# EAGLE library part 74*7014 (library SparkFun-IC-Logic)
Schmitt-trigger Hex Buffer The 74HC7014 is a hex buffer with precision Schmitt-trigger inputs. The precisely defined trigger levels are lying in a window between (0.55 x VCC) and (0.65 x VCC). It makes the circuit suitable to operate in a highly noisy environment. Input shorts are allowed to -1.5 V and +16 V without disturbing other channels. Inputs include clamp diodes that enable the use of current limiting resistors to interface inputs to voltages in excess of VCC. Schmitt trigger inputs transform slowly changing input signals into sharply defined jitter-free output signals. SparkFun Products SparkFun Stepoko (ROB-13899)
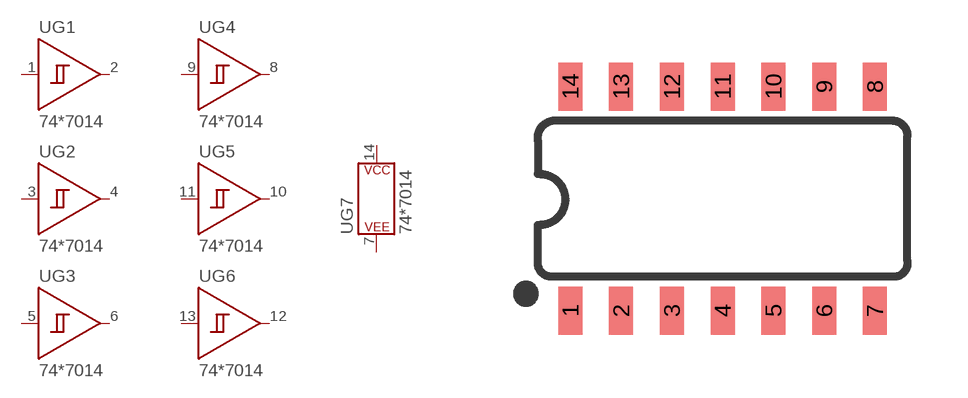
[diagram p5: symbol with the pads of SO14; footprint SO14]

Designator prefix U; gates G1=GATE_INVERTER_SCHMITT_TRIGGER G2=GATE_INVERTER_SCHMITT_TRIGGER G3=GATE_INVERTER_SCHMITT_TRIGGER G4=GATE_INVERTER_SCHMITT_TRIGGER G5=GATE_INVERTER_SCHMITT_TRIGGER G6=GATE_INVERTER_SCHMITT_TRIGGER G7=POWER_CONSORT

## 74HC7014D (PROD_ID: IC-12527; VALUE: 74HC7014D)  [SO14]
1  G1:A
2  G1:Y
3  G2:A
4  G2:Y
5  G3:A
6  G3:Y
7  G7:P$V-
8  G4:Y
9  G4:A
10  G5:Y
11  G5:A
12  G6:Y
13  G6:A
14  G7:P$V+

## Footprint SO14 (pad centres in mm)
SOIC, 0.15 inch width
smd 0.6 x 1.2: 1 -3.175,-2.8; 2 -1.905,-2.8; 3 -0.635,-2.8; 4 0.635,-2.8; 5 1.905,-2.8; 6 3.175,-2.8; 7 4.445,-2.8; 8 4.445,2.8; 9 3.175,2.8; 10 1.905,2.8; 11 0.635,2.8; 12 -0.635,2.8; 13 -1.905,2.8; 14 -3.175,2.8

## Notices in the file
Licensing: Creative Commons ShareAlike 4.0 International - https://creativecommons.org/licenses/by-sa/4.0
